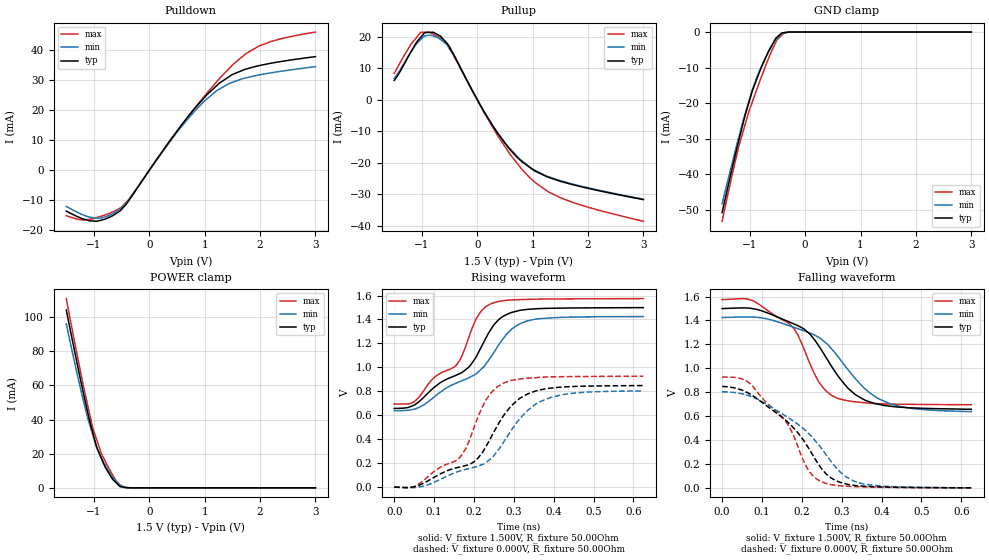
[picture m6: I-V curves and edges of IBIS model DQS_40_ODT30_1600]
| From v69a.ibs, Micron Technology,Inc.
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| MODEL DQS_40_ODT30_1600 (40 Ohm Data Strobe I/O with 30ohm ODT, 1600Mbps)
[Model]   DQS_40_ODT30_1600
Model_type   I/O
Vinl = 600.000mV
Vinh = 900.000mV
Vmeas = 750.000mV
Vref = 750.000mV
Cref = 0.0pF
Rref = 25.000Ohm
|   typ   min   max
C_comp   1.22pF   1.07pF   1.39pF
| Note: C_comp changes when the ODT circuit is enabled.
[Model Spec]
| Input threshold voltage corners
Vinl   0.6000V   0.5625V   0.6375V
Vinh   0.9000V   0.8625V   0.9375V
| Measurement voltage corners
Vmeas   0.7500V   0.7125V   0.7875V
| Timing spec test load voltage corners
Vref   0.7500V   0.7125V   0.7875V
|[Receiver Thresholds]
|Vth   =  0.750V
|Vth_min  =  0.735V
|Vth_max  =  0.765V
|Vinh_ac  =  0.150V
|Vinh_dc  =  0.100V
|Vinl_ac  = -0.150V
|Vinl_dc  = -0.100V
|Tslew_ac =  5.000ns |Not specified, so set to high value
|Threshold_sensitivity = 0.50
|Reference_supply Pullup_ref
[Receiver Thresholds]
Vcross_low   = 0.600V
Vcross_high  = 0.900V
Vdiff_ac   = 300mV
Vdiff_dc   = 200mV
Tdiffslew_ac = 10.000ns |Not specified, so set to high value
[Voltage Range]   1.5000V   1.4250V   1.5750V
[Pullup Reference]   1.5000V   1.4250V   1.5750V
| Junction Temperature (Ambient temp is 35C typ, 95C min, 0C max)
[Temperature Range]   50.0   110.0   0.0
[Add Submodel]
| Submodel Name   Mode
30ohm_ODT_1600   Non-Driving
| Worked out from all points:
|   slope of the pulldown table from 0 to 0.225 V, typ, clamps not added: 37.3 ohm
|   slope of the pullup table from 0 to 0.225 V, typ, clamps not added: 33.3 ohm
|   GND clamp passes 1 mA (typ) near -0.48 V on its own axis
|   POWER clamp passes 1 mA (typ) near -0.54 V on its own axis
|   falling waveform, V_fixture 1.500V, R_fixture 50.00Ohm: 20-80 % time 114ps typ, 133ps min, 90.6ps max; typ from 1.5 V to 0.657 V
|   rising waveform, V_fixture 1.500V, R_fixture 50.00Ohm: 20-80 % time 148ps typ, 163ps min, 117ps max; typ from 0.657 V to 1.5 V
|   rising waveform, V_fixture 0.000V, R_fixture 50.00Ohm: 20-80 % time 127ps typ, 142ps min, 105ps max; typ from 0 V to 0.848 V
|   falling waveform, V_fixture 0.000V, R_fixture 50.00Ohm: 20-80 % time 133ps typ, 149ps min, 107ps max; typ from 0.848 V to 0 V
[Pulldown]
|   Voltage   I(typ)   I(min)   I(max)
-1.5V     -13.6mA    -12.02mA   -15.12mA
-1.195V   -16.21mA   -14.86mA   -16.58mA
-965mV    -16.97mA   -15.99mA   -15.86mA
-800mV    -16.27mA   -15.52mA   -14.88mA
-530mV    -13.56mA   -12.95mA   -12.57mA
-380mV    -10.33mA   -10.03mA   -9.938mA
300mV     7.984mA    7.783mA    7.776mA
755mV     19.11mA    18.35mA    19.04mA
1.215V    28.11mA    26.43mA    29.39mA
1.49V     31.72mA    29.18mA    34.78mA
1.975V    34.76mA    31.65mA    41.24mA
3V        37.78mA    34.43mA    45.95mA
[GND Clamp]
|   Voltage   I(typ)   I(min)   I(max)
-1.5V     -50.86mA   -48.39mA   -53.31mA
-1.32V    -38.49mA   -36.95mA   -40.31mA
-1.195V   -30.28mA   -29.36mA   -32mA
-1.09V    -23.76mA   -23.33mA   -26.33mA
-950mV    -16.36mA   -16.11mA   -19.5mA
-810mV    -10.64mA   -10.39mA   -13.44mA
-660mV    -5.343mA   -5.541mA   -7.383mA
-550mV    -2.294mA   -2.517mA   -3.532mA
-505mV    -1.389mA   -1.77mA    -2.13mA
-430mV    -374uA     -539.4uA   -960.1uA
-380mV    -171.4uA   -317.5uA   -180.2uA
3V        0A         0A         0A
[Pullup]
|   Voltage   I(typ)   I(min)   I(max)
-1.5V     6.153mA    6.805mA    8.388mA
-1.2V     15.14mA    15.12mA    17.57mA
-1.025V   19.77mA    19.04mA    21.32mA
-950mV    21.3mA     20.21mA    21.45mA
-795mV    21.44mA    20.27mA    20.85mA
-660mV    20.15mA    19.1mA     19.54mA
-505mV    16.8mA     16.28mA    16.93mA
345mV     -10.07mA   -9.849mA   -10.68mA
805mV     -19.63mA   -19.32mA   -22mA
1.055V    -22.71mA   -22.45mA   -26.38mA
1.51V     -25.9mA    -25.71mA   -31.14mA
3V        -31.67mA   -31.54mA   -38.55mA
[POWER Clamp]
|   Voltage   I(typ)   I(min)   I(max)
-1.5V     104.2mA    96.04mA    110.8mA
-1.195V   56.08mA    51.65mA    60.2mA
-1.11V    43.68mA    40.43mA    47.85mA
-1.025V   32.84mA    31.3mA     35.51mA
-950mV    23.76mA    23.64mA    28.1mA
-870mV    17.62mA    17.65mA    20.38mA
-795mV    11.95mA    13.1mA     15.38mA
-665mV    5.081mA    6.451mA    7.641mA
-550mV    1.395mA    1.908mA    2.415mA
-505mV    588.2uA    1.278mA    931.8uA
-315mV    8.745uA    20.93uA    7.341uA
3V        0A         0A         0A
[Ramp]
R_load = 50.00Ohm
|   typ   min   max
dV/dt_r   508.798mV/127.180ps 481.925mV/142.095ps 555.841mV/105.459ps
dV/dt_f   504.967mV/113.872ps 472.002mV/132.514ps 527.439mV/90.594ps
[Falling Waveform]
V_fixture = 1.500V
V_fixture_min = 1.425V
V_fixture_max = 1.575V
R_fixture = 50.00Ohm
|   Time   V(typ)   V(min)   V(max)
0s        1.499V     1.424V     1.574V
75ps      1.499V     1.429V     1.567V
170ps     1.385V     1.354V     1.366V
190ps     1.356V     1.331V     1.278V
245ps     1.174V     1.254V     874.4mV
290ps     938.4mV    1.1V       748.1mV
335ps     777.5mV    910.3mV    718.9mV
370ps     719.1mV    795.2mV    707.4mV
420ps     683.5mV    704.5mV    701.2mV
625ps     657.2mV    637.7mV    695.1mV
[Rising Waveform]
V_fixture = 1.500V
V_fixture_min = 1.425V
V_fixture_max = 1.575V
R_fixture = 50.00Ohm
|   Time   V(typ)   V(min)   V(max)
0s        657.2mV    637.7mV    695.1mV
50ps      684.7mV    651mV      712.6mV
105ps     845.5mV    765.7mV    928.4mV
155ps     933.8mV    868.6mV    1.015V
190ps     1.012V     917.1mV    1.278V
210ps     1.116V     959.6mV    1.429V
245ps     1.33V      1.099V     1.534V
295ps     1.459V     1.32V      1.563V
335ps     1.485V     1.389V     1.568V
625ps     1.499V     1.424V     1.574V
[Rising Waveform]
V_fixture = 0.000V
V_fixture_min = 0.000V
V_fixture_max = 0.000V
R_fixture = 50.00Ohm
|   Time   V(typ)   V(min)   V(max)
0s        250uV      145.9uV    134.6uV
50ps      2.797mV    -3.377mV   4.784mV
165ps     168.6mV    135.2mV    249.9mV
180ps     180.9mV    149.4mV    325.6mV
205ps     222.2mV    169.8mV    541.2mV
230ps     338.3mV    205mV      727.4mV
275ps     600.6mV    378.9mV    870.6mV
330ps     770.3mV    626mV      908.8mV
390ps     825.7mV    746mV      920.1mV
625ps     848.2mV    803.4mV    926.5mV
[Falling Waveform]
V_fixture = 0.000V
V_fixture_min = 0.000V
V_fixture_max = 0.000V
R_fixture = 50.00Ohm
|   Time   V(typ)   V(min)   V(max)
0s        848.2mV    803.4mV    926.5mV
60ps      802.2mV    778.1mV    896.1mV
150ps     590.9mV    620mV      594.2mV
175ps     516.1mV    566.7mV    467.4mV
215ps     342.1mV    460.1mV    156.1mV
245ps     181.5mV    349mV      57.6mV
265ps     103.5mV    258mV      33.37mV
295ps     47.17mV    135.5mV    17.66mV
350ps     15.12mV    36.06mV    8.58mV
625ps     250uV      145.9uV    134.6uV
